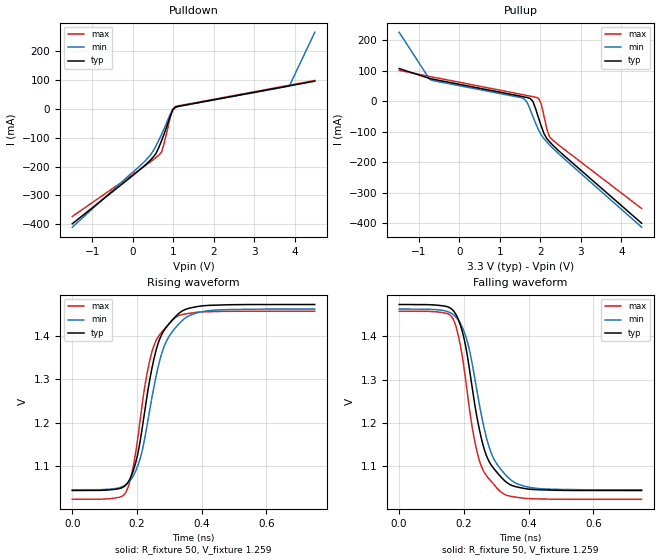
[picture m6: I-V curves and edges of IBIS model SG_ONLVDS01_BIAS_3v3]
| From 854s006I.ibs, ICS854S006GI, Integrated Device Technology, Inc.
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[Model] SG_ONLVDS01_BIAS_3v3
Model_type   Output
Polarity   Non-Inverting
|   typ   min   max
C_comp   2pF   1.5pF   2.5pF
Vmeas = 1.259V
Rref = 50
Cref = 0
Vref = 1.295V
|   typ   min   max
[Voltage range]   3.3V   3.135V   3.465V
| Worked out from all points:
|   slope of the pulldown table from 0 to 0.495 V, typ, clamps not added: 8 ohm
|   slope of the pullup table from 0 to 0.495 V, typ, clamps not added: 38.7 ohm
|   rising waveform, R_fixture 50, V_fixture 1.259: 20-80 % time 64.3ps typ, 71.6ps min, 57.9ps max; typ from 1.04 V to 1.47 V
|   falling waveform, R_fixture 50, V_fixture 1.259: 20-80 % time 64.3ps typ, 71.6ps min, 57.9ps max; typ from 1.47 V to 1.04 V
[Pulldown]
|Voltage   I (typ)   I (min)   I (max)
-1.49V    -397.8mA   -409.5mA   -372.5mA
300.1mV   -196.1mA   -181.6mA   -197.9mA
437.8mV   -178.1mA   -160.5mA   -183.8mA
575.5mV   -155.4mA   -128.9mA   -168.9mA
713.2mV   -111.5mA   -89.68mA   -150.8mA
782.1mV   -86.04mA   -68.01mA   -117.8mA
919.8mV   -29.81mA   -21.87mA   -35.73mA
988.6mV   -5.188mA   -3.331mA   -1.665mA
1.057V    5.313mA    4.977mA    7.676mA
3.743V    75.82mA    75.18mA    77.96mA
3.88V     79.38mA    80.93mA    81.55mA
4.5V      95.42mA    264.3mA    97.68mA
[Pullup]
|Voltage   I (typ)   I (min)   I (max)
-1.49V    107.6mA    226.6mA    101.7mA
-732.6mV  74.83mA    71.52mA    81.64mA
1.539V    16.03mA    11.35mA    22.49mA
1.677V    12.39mA    -5.314mA   18.9mA
1.746V    9.581mA    -26.63mA   17.11mA
1.815V    -777.1uA   -50.05mA   15.31mA
1.953V    -54.13mA   -93.62mA   10.17mA
2.021V    -81.68mA   -110.8mA   -9.106mA
2.09V     -106.9mA   -123.1mA   -49.54mA
2.159V    -122.3mA   -133.7mA   -91.33mA
2.228V    -133.1mA   -143.4mA   -117.5mA
4.5V      -400.4mA   -413.3mA   -352.1mA
[Ramp]
|   typ   min   max
dV/dt_r   0.342/0.113n   0.333/0.125n   0.346/0.103n
dV/dt_f   0.342/0.113n   0.333/0.125n   0.346/0.103n
R_load =   50.0000
[Rising Waveform]
R_fixture = 50
V_fixture   =1.259   |Vcc_typ
V_fixture_min=1.25406  |Vcc_min
V_fixture_max=1.24065  |Vcc_max
C_fixture = 0.0p
| Time   typ   min   max
0s        1.044V     1.046V     1.024V
165.9ps   1.057V     1.058V     1.041V
183.2ps   1.079V     1.072V     1.081V
201.2ps   1.125V     1.099V     1.158V
224.5ps   1.231V     1.167V     1.286V
245.5ps   1.323V     1.256V     1.362V
278.5ps   1.407V     1.365V     1.411V
316.1ps   1.443V     1.417V     1.441V
415.2ps   1.471V     1.458V     1.456V
749.2ps   1.473V     1.462V     1.457V
[Falling Waveform]
R_fixture = 50
V_fixture   =1.259   |Vcc_typ
V_fixture_min=1.25406  |Vcc_min
V_fixture_max=1.24065  |Vcc_max
C_fixture = 0.0p
| Time   typ   min   max
0s        1.473V     1.462V     1.457V
165.9ps   1.46V      1.45V      1.441V
183.2ps   1.438V     1.437V     1.4V
201.2ps   1.392V     1.41V      1.323V
224.5ps   1.286V     1.341V     1.196V
245.5ps   1.194V     1.252V     1.12V
278.5ps   1.11V      1.143V     1.07V
316.1ps   1.074V     1.091V     1.04V
415.2ps   1.046V     1.05V      1.025V
749.2ps   1.044V     1.046V     1.024V
